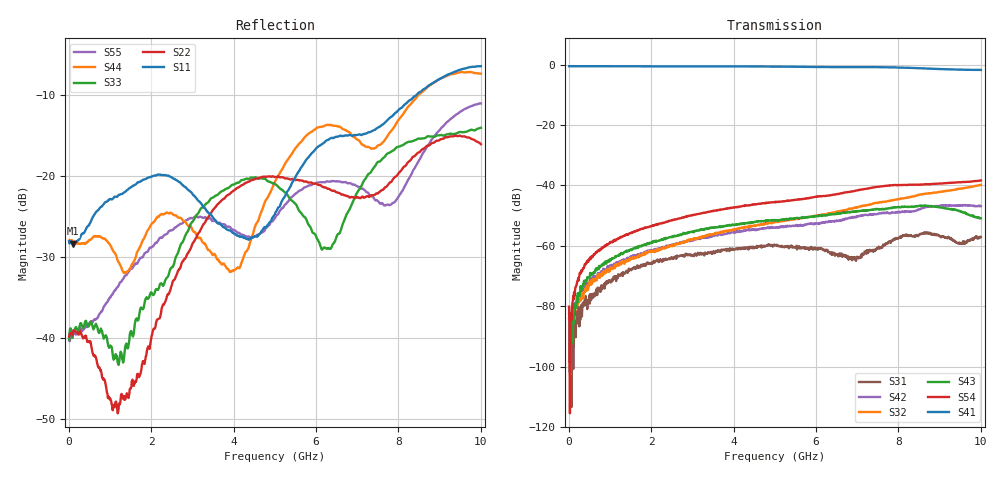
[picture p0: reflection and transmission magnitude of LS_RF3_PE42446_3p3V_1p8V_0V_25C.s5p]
! Created Wed Jan 31 17:41:41 2024
# ghz S ma R 50
! 5 Port Network Data from SP1.SP block
! freq  magS11  angS11  magS12  angS12  magS13  angS13  magS14  angS14
!  magS15  angS15
!  magS21  angS21  magS22  angS22  magS23  angS23
!  magS24  angS24  magS25  angS25
!  magS31  angS31  magS32  angS32
!  magS33  angS33  magS34  angS34  magS35  angS35
!  magS41  angS41
!  magS42  angS42  magS43  angS43  magS44  angS44  magS45  angS45
!  magS51  angS51  magS52  angS52  magS53  angS53  magS54  angS54
!  magS55  angS55
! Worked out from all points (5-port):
!   1000 points, 10 MHz to 10 GHz, reference 50 ohm
!   strongest paths, dB at 10 MHz, 2.51 GHz, 5.01 GHz, 7.51 GHz, 10 GHz:
!     S41: -0.5, -0.6, -0.7, -0.9, -1.8
!     S54: -80.1, -51.6, -45.6, -40.4, -38.4
!     S43: -82.6, -57.2, -51.5, -47.8, -50.9
!     S32: -98.2, -60.1, -52.0, -45.7, -39.8
!     S42: -84.2, -59.6, -53.9, -49.4, -46.8
!     S31: -80.7, -63.9, -59.8, -60.8, -57.1
!   lowest |S11| = -28.4 dB at 110 MHz (marker M1), VSWR 1.08, Z = 54 - j0.0169 ohm
!   |S11| at or under -10 dB: start of sweep to 8.446 GHz
